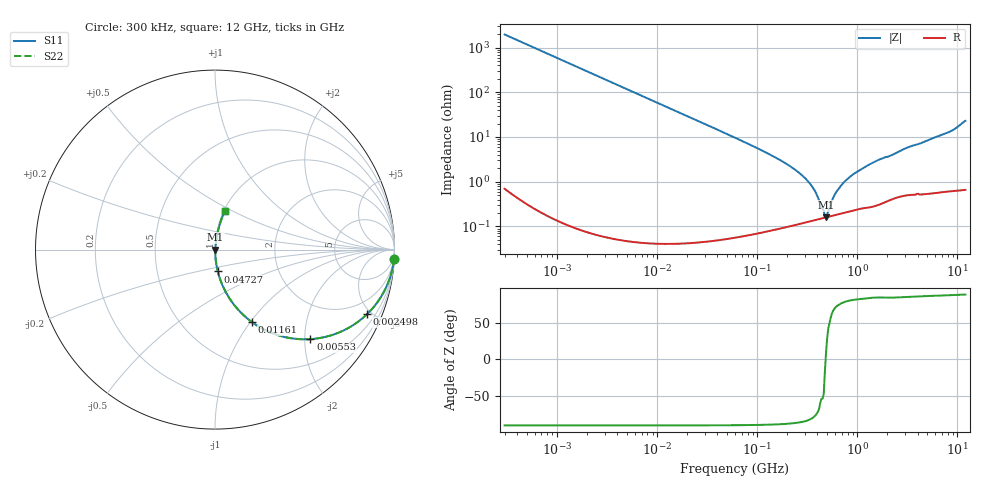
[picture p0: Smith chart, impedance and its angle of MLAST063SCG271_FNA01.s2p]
! MLAST063SCG271_FNA01  S-PARAMETER MODEL  ( General Type )
! Model Generated by TAIYO YUDEN Corporation (http://www.ty-top.com)
! Version 1.0
! TAIYO YUDEN Control No. 160830
! Copyright(c) 2016 TAIYO YUDEN CO.,LTD. All Rights Reserved.
! Product Description (link to TY-COMPAS)
! https://ds.yuden.co.jp/TYCOMPAS/or/detail?pn=MLAST063SCG271JFNA01&u=M
! Products Name : Multilayer Ceramic Capacitors
! Characteristics :
!  Capacitance : 270 pF , Rated Voltage : 25V , TCC : CG / C0G
!  Case Size : 0.6 x 0.3 / 0.024 x 0.012 [mm/inch] , Thickness : 0.3 / 0.012 [mm/inch]
!  (Conditions: Temperature = 25 degC , DC Bias Current/Voltage = 0A / 0V)
! External Node Assignments :
!  1  o---| |---o  2
! GND o---------o GND
! Frequency Range : 0.3MHz  -  12000MHz  [ 401 STEP ]
# MHz S RI R 50
! Freq[MHz].  S11 Real  S11 Imag  S21 Real  S21 Imag  S12 Real  S12 Imag  S22 Real  S22 Imag
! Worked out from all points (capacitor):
!   401 points, 300 kHz to 12 GHz, reference 50 ohm
!   read as one part in series: C = 270 pF near 316.3 kHz
!   lowest |Z| = 162 mohm at 486.5 MHz (marker M1)
!   series resonance near 482.4 MHz, so ESL is about 400 pH
!   S11 on the Smith chart (normalised r, x): 300 kHz: 1, -39; 2.498 MHz: 1.00, -4.72; 5.53 MHz: 1.00, -2.13; 11.61 MHz: 1.00, -1.01; 47.27 MHz: 1.00, -0.25; 12 GHz: 1.01, +0.46
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0.3  0.9974 -0.0508  0.0026 0.0508  0.0026 0.0508  0.9974 -0.0508
0.778586  0.9828 -0.1298  0.0172 0.1298  0.0172 0.1298  0.9828 -0.1298
1.769972  0.9172 -0.2754  0.0828 0.2754  0.0828 0.2754  0.9172 -0.2754
2.49766  0.8477 -0.3592  0.1523 0.3592  0.1523 0.3592  0.8477 -0.3592
5.529524  0.5318 -0.4988  0.4682 0.4988  0.4682 0.4988  0.5318 -0.4988
10.44266  0.2416 -0.4277  0.7584 0.4277  0.7584 0.4277  0.2416 -0.4277
11.60999  0.205 -0.4033  0.795 0.4033  0.795 0.4033  0.205 -0.4033
20.79434  0.0745 -0.2618  0.9255 0.2618  0.9255 0.2618  0.0745 -0.2618
47.2721  0.0155 -0.1215  0.9845 0.1215  0.9845 0.1215  0.0155 -0.1215
60  0.00981 -0.0957  0.9902 0.0957  0.9902 0.0957  0.00981 -0.0957
202.9496  0.00155 -0.0238  0.9984 0.0238  0.9984 0.0238  0.00155 -0.0238
278.9009  0.00137 -0.014  0.9986 0.014  0.9986 0.014  0.00137 -0.014
353.9943  0.00139 -0.00766  0.9986 0.00766  0.9986 0.00766  0.00139 -0.00766
461.3684  0.00155 -0.00168  0.9984 0.00168  0.9984 0.00168  0.00155 -0.00168
486.4723  0.0016 0.000231  0.9984 -0.000231  0.9984 -0.000231  0.0016 0.000231
512.9422  0.00165 0.00151  0.9984 -0.00151  0.9984 -0.00151  0.00165 0.00151
601.3112  0.00183 0.00507  0.9982 -0.00507  0.9982 -0.00507  0.00183 0.00507
783.7017  0.00221 0.0109  0.9978 -0.0109  0.9978 -0.0109  0.00221 0.0109
1331.232  0.00327 0.0244  0.9967 -0.0244  0.9967 -0.0244  0.00327 0.0244
2088.533  0.00518 0.0369  0.9948 -0.0369  0.9948 -0.0369  0.00518 0.0369
8281.503  0.0222 0.1259  0.9778 -0.1259  0.9778 -0.1259  0.0222 0.1259
12000  0.0558 0.2156  0.9442 -0.2156  0.9442 -0.2156  0.0558 0.2156
